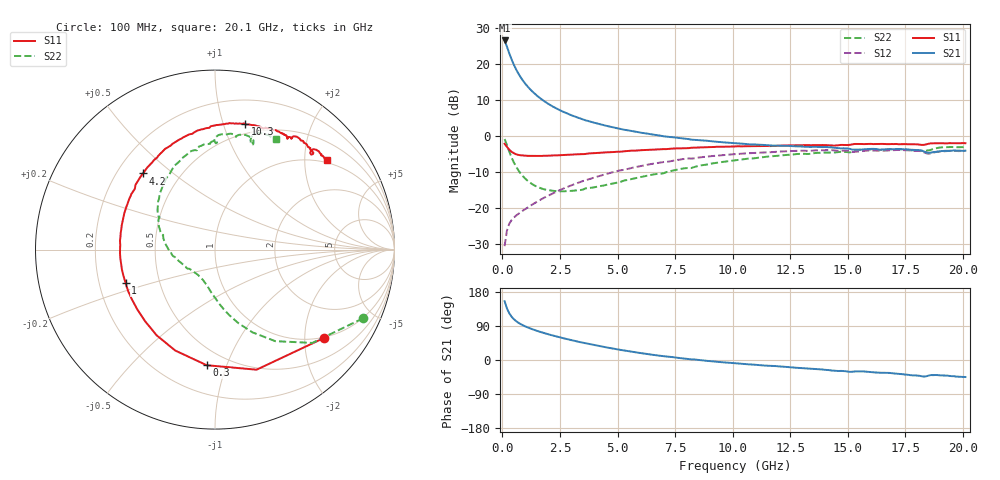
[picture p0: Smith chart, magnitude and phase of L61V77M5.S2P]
!  Infineon Technologies AG
! BFR380L3 , PF131585-7, No.6, Th 09.10.01, soldered on pcb-board, measured with PP GSG850
!  Vce=1.75 V,  Ic=7.5 mA
! Common Emitter S-Parameters:  15. November 2001
#  GHz  S  MA  R  50
! f  S11  S21  S12  S22
! GHz  Mag  Ang  Mag  Ang  Mag  Ang  Mag  Ang
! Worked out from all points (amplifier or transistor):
!   201 points, 100 MHz to 20.1 GHz, reference 50 ohm
!   highest |S21| = 26.7 dB at 100 MHz (marker M1)
!   |S21| within 3 dB of that: start of sweep to 270.2 MHz
!   unconditionally stable (mu >= 1): 1.967 GHz to 4.788 GHz
!   at 3.4 GHz: K = 1.04, MAG = 7.6 dB, |S12| = -12.8 dB
!   at 10.1 GHz: K = 0.96, MSG = 1.5 dB, |S12| = -5.0 dB
!   at 20.1 GHz: K = 0.99, MSG = 0.0 dB, |S12| = -4.1 dB
!   S11 on the Smith chart (normalised r, x): 100 MHz: 0.98, -2.49; 300 MHz: 0.39, -0.85; 1 GHz: 0.31, -0.16; 4.2 GHz: 0.31, +0.40; 10.3 GHz: 0.41, +1.18; 20.1 GHz: 0.94, +2.55
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0.1  0.7821 -39.0  21.51 155.2  0.02922 68.8  0.9087 -24.9
0.2  0.708 -70.9  17.67 136.3  0.04817 58.3  0.7513 -43.8
0.3  0.6459 -94.1  14.3 123.5  0.05992 51.1  0.6108 -56.6
0.4  0.6044 -111.5  11.76 114.4  0.06737 47.2  0.5059 -65.7
0.5  0.5777 -124.3  9.877 107.7  0.07301 45.7  0.43 -72.4
0.6  0.5576 -134.3  8.472 102.5  0.07812 45.5  0.3747 -77.6
0.7  0.5463 -142.4  7.413 98.2  0.08247 45.6  0.3323 -82.1
0.8  0.5397 -149.2  6.573 94.5  0.08714 46.3  0.2998 -85.9
1  0.5317 -159.5  5.358 88.5  0.09636 47.6  0.2543 -92.2
1.2  0.5304 -167.8  4.521 83.5  0.1061 49.2  0.2247 -97.8
1.4  0.5296 -174.5  3.915 79.1  0.1162 50.5  0.2047 -102.8
1.9  0.5316 172.2  2.946 69.6  0.1428 52.6  0.1785 -113.9
2.6  0.5444 158.1  2.214 58.2  0.1825 53.1  0.1702 -128.2
3.5  0.5602 143.1  1.706 45.6  0.2364 51.1  0.1795 -143.6
4.2  0.5839 133.4  1.473 37.0  0.2769 48.5  0.1995 -156.5
5.2  0.6095 121.5  1.241 25.9  0.3355 42.7  0.2345 -170.8
6.8  0.6547 103.7  1.021 11.5  0.426 33.3  0.2991 165.3
10.1  0.7166 77.9  0.7938 -8.6  0.5593 11.8  0.46 129.2
10.3  0.7197 76.5  0.7881 -9.5  0.5658 10.5  0.4677 127.1
13.5  0.7469 60.0  0.7091 -23.3  0.6283 -9.5  0.5748 99.5
16.8  0.7718 47.7  0.6564 -34.1  0.6313 -25.7  0.6556 77.5
20.1  0.7956 38.6  0.6265 -44.9  0.6229 -39.3  0.7045 61.0
